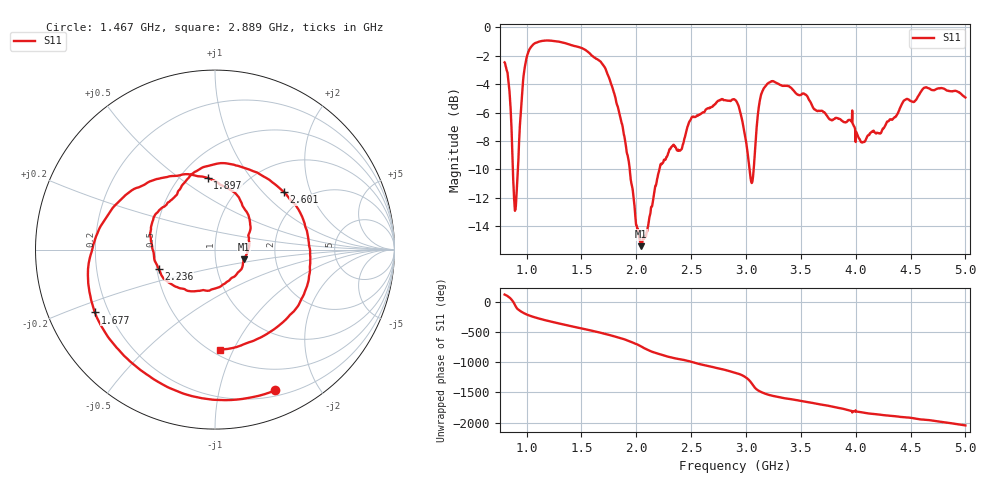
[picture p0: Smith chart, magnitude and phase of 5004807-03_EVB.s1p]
#  HZ  S  RI  R  50.00
! Rohde & Schwarz ZVA/B
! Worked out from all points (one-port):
!   1601 points, 800 MHz to 5 GHz, reference 50 ohm
!   lowest |S11| = -15.4 dB at 2.044 GHz (marker M1), VSWR 1.41, Z = 68.7 - j7.59 ohm
!   |S11| at or under -10 dB: 875.3 MHz to 921.5 MHz (46.18 MHz wide, 5.14 % of centre); 1.94 GHz to 2.21 GHz (270 MHz wide, 13 % of centre); 3.033 GHz to 3.07 GHz (37.37 MHz wide, 1.22 % of centre)
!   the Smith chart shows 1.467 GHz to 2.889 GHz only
!   S11 on the Smith chart (normalised r, x): 1.467 GHz: 0.26, -1.48; 1.677 GHz: 0.15, -0.24; 1.897 GHz: 0.67, +0.64; 2.236 GHz: 0.51, -0.13; 2.601 GHz: 1.55, +1.33; 2.889 GHz: 0.55, -0.89
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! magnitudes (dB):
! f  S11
! 800 MHz  -2.5
! 839.4 MHz  -4.1
! 884 MHz  -11.7
! 899.8 MHz  -12.8
! 965.4 MHz  -4.0
! 1.013 GHz  -1.8
! 1.325 GHz  -1.1
! 1.467 GHz  -1.4
! 1.677 GHz  -2.4
! 1.85 GHz  -6.2
! 1.897 GHz  -7.9
! 2.044 GHz  -15.4
! 2.091 GHz  -14.6
! 2.236 GHz  -9.6
! 2.375 GHz  -8.7
! 2.601 GHz  -6.0
! 2.889 GHz  -5.1
! 2.9 GHz  -5.1
! 2.96 GHz  -6.4
! 3.052 GHz  -11.0
! 3.118 GHz  -5.6
! 3.157 GHz  -4.4
! 3.425 GHz  -4.4
! 3.95 GHz  -6.5
! 4.068 GHz  -8.1
! 4.475 GHz  -5.1
! 4.638 GHz  -4.2
! 5 GHz  -4.9
